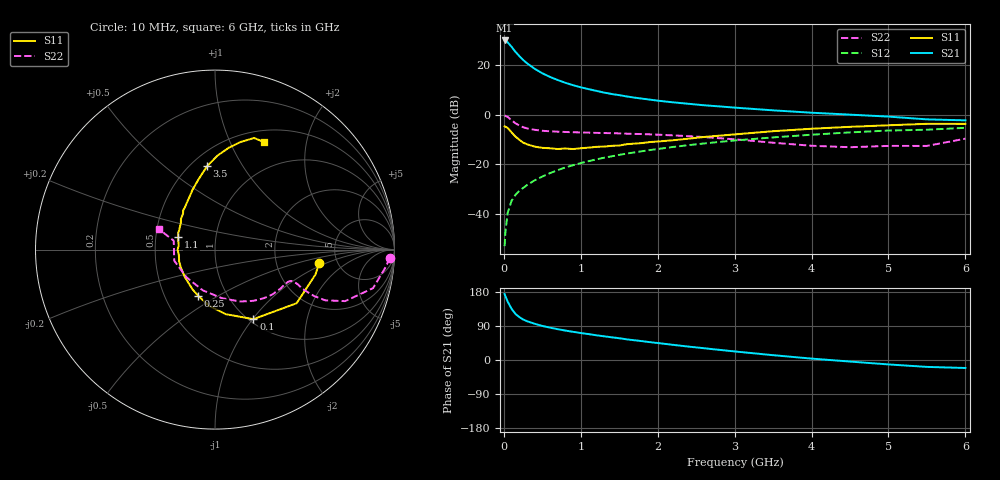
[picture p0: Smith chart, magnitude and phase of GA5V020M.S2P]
! Infineon Technologies  Discrete & RF Semiconductors
! BF775
! Si NPN RF Bipolar Junction Transistor in SOT23
! VCE = 5 V  IC = 20 mA
! Common Emitter S-Parameters:  May  1996
# GHz  S  MA  R  50
!  f  S11  S21  S12  S22
! GHz  MAG  ANG  MAG  ANG  MAG  ANG  MAG  ANG
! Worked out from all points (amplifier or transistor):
!   36 points, 10 MHz to 6 GHz, reference 50 ohm
!   highest |S21| = 30.1 dB at 10 MHz (marker M1)
!   |S21| within 3 dB of that: start of sweep to 111.3 MHz
!   unconditionally stable (mu >= 1): 420.7 MHz to 2.862 GHz
!   at 250 MHz: K = 0.86, MSG = 25.9 dB, |S12| = -29.6 dB
!   at 1.4 GHz: K = 1.10, MAG = 10.7 dB, |S12| = -16.8 dB
!   at 6 GHz: K = 0.93, MSG = 1.5 dB, |S12| = -5.2 dB
!   S11 on the Smith chart (normalised r, x): 10 MHz: 3.61, -0.84; 100 MHz: 1.05, -1.01; 250 MHz: 0.73, -0.41; 1.1 GHz: 0.65, +0.10; 3.5 GHz: 0.60, +0.71; 6 GHz: 0.64, +1.35
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0.01  0.5853 -7.5  32.04 174.1  0.0022 88.4  0.9746 -2.7
0.02  0.5768 -13.9  31.59 168.7  0.0042 83.8  0.9562 -5.8
0.05  0.5442 -33.3  29.37 154.1  0.0104 76.6  0.9065 -13.7
0.1  0.4427 -61.1  23.89 135.2  0.0182 70.3  0.7798 -21.6
0.15  0.3643 -80.7  19 121.9  0.024 66.0  0.6764 -24.7
0.2  0.3142 -96.3  15.57 113.4  0.0288 66.9  0.6095 -25.1
0.25  0.2744 -109.8  12.96 107.0  0.0331 66.8  0.563 -24.6
0.3  0.2544 -119.5  11.09 102.4  0.0379 68.1  0.533 -24.1
0.4  0.2274 -137.5  8.582 95.7  0.0473 69.3  0.4984 -22.7
0.5  0.2152 -151.4  6.939 89.9  0.0564 70.0  0.476 -22.2
0.6  0.2108 -161.3  5.855 85.4  0.0662 70.5  0.4654 -22.2
0.7  0.2036 -171.7  5.072 81.3  0.0761 70.7  0.4567 -22.5
0.8  0.2083 -179.8  4.452 77.7  0.0862 70.1  0.4505 -23.1
0.9  0.2033 173.1  3.981 74.3  0.0959 69.8  0.4444 -23.9
1.1  0.217 160.7  3.319 68.4  0.1154 68.7  0.4368 -26.3
1.3  0.228 150.4  2.831 62.6  0.1353 67.1  0.4287 -28.7
1.6  0.2554 138.0  2.353 54.4  0.1646 64.4  0.416 -33.4
2.2  0.3061 120.6  1.791 40.0  0.224 58.4  0.3843 -44.6
3.5  0.4669 95.4  1.234 12.7  0.3497 42.9  0.2728 -82.1
4.5  0.5726 82.3  1.01 -4.1  0.4415 29.8  0.2214 -135.9
5.5  0.6589 70.7  0.81 -18.2  0.4999 14.6  0.2352 167.9
6  0.6584 65.6  0.774 -21.1  0.5465 10.3  0.3296 160.1
